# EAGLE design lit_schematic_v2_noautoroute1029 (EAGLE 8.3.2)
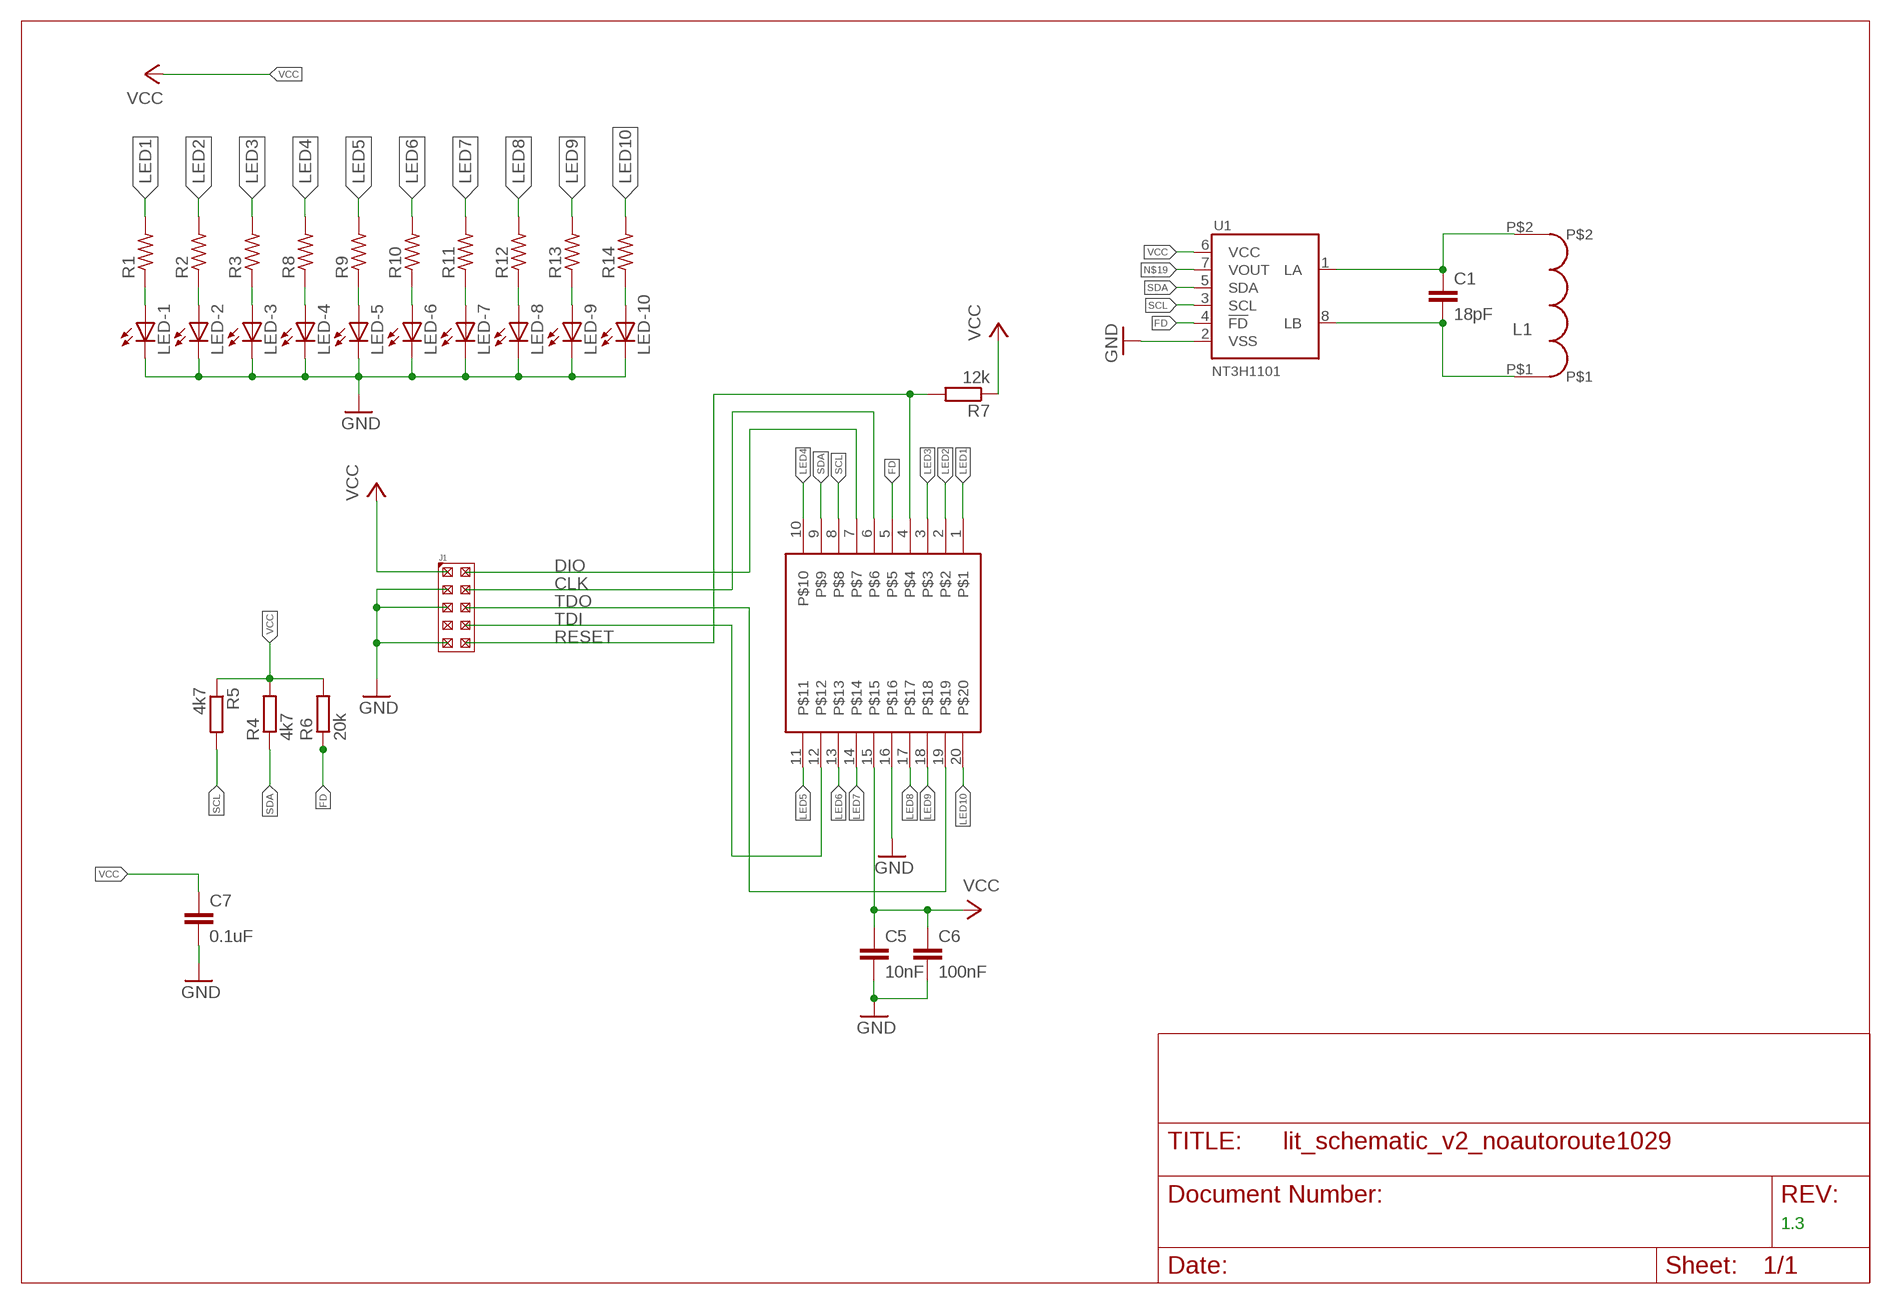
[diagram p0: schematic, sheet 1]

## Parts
C1  18pF  C-EUC0402K  [C0402K]
C5  10nF  C-EUC0402K  [C0402K]
C6  100nF  C-EUC0402K  [C0402K]
C7  0.1uF  C-EUC0402K  [C0402K]
J1  J-10-2X5_B0D95-10  [BD095-10]
L1  NXP_PICC_ANTENNAS_TEST_CLASS_05_50PF_01  [NXP_PICC_ANTENNAS_TEST_L_PICC_CLASS5_50PF_01]
LED-1  LEDCHIPLED_1206  [CHIPLED_1206]
LED-2  LEDCHIPLED_1206  [CHIPLED_1206]
LED-3  LEDCHIPLED_1206  [CHIPLED_1206]
LED-4  LEDCHIPLED_1206  [CHIPLED_1206]
LED-5  LEDCHIPLED_1206  [CHIPLED_1206]
LED-6  LEDCHIPLED_1206  [CHIPLED_1206]
LED-7  LEDCHIPLED_1206  [CHIPLED_1206]
LED-8  LEDCHIPLED_1206  [CHIPLED_1206]
LED-9  LEDCHIPLED_1206  [CHIPLED_1206]
LED-10  LEDCHIPLED_1206  [CHIPLED_1206]
R1  R-US_R0402  [R0402]
R2  R-US_R0402  [R0402]
R3  R-US_R0402  [R0402]
R4  4k7  R-EU_R0402  [R0402]
R5  4k7  R-EU_R0402  [R0402]
R6  20k  R-EU_R0402  [R0402]
R7  12k  R-EU_R0402  [R0402]
R8  R-US_R0402  [R0402]
R9  R-US_R0402  [R0402]
R10  R-US_R0402  [R0402]
R11  R-US_R0402  [R0402]
R12  R-US_R0402  [R0402]
R13  R-US_R0402  [R0402]
R14  R-US_R0402  [R0402]
U1  NT3H1101  [TSSOP8]
U$1  LPC812  NXP_LPC80012_TSSOP20  [TSSOP20]

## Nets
CLK: J1.P$4 U$1.6
DIO: J1.P$2 U$1.7
FD: R6.1 U1.4(!FD) U$1.5
GND: C5.2 C6.2 C7.2 J1.P$3 J1.P$5 J1.P$9 LED-1.C LED-2.C LED-3.C LED-4.C LED-5.C LED-6.C LED-7.C LED-8.C LED-9.C LED-10.C U1.2(VSS) U$1.16
LED1: R1.2 U$1.1
LED2: R2.2 U$1.2
LED3: R3.2 U$1.3
LED4: R8.2 U$1.10
LED5: R9.2 U$1.11
LED6: R10.2 U$1.13
LED7: R11.2 U$1.14
LED8: R12.2 U$1.17
LED9: R13.2 U$1.18
LED10: R14.2 U$1.20
N$1: C1.2 L1.P$1 U1.8(LB)
N$2: LED-1.A R1.1
N$3: LED-2.A R2.1
N$4: LED-3.A R3.1
N$5: LED-4.A R8.1
N$6: LED-5.A R9.1
N$7: LED-6.A R10.1
N$8: LED-7.A R11.1
N$9: LED-8.A R12.1
N$10: LED-9.A R13.1
N$13: C1.1 L1.P$2 U1.1(LA)
N$15: LED-10.A R14.1
N$19: U1.7(VOUT)
RESET: J1.P$10 R7.2 U$1.4
SCL: R5.2 U1.3(SCL) U$1.8
SDA: R4.1 U1.5(SDA) U$1.9
TDI: J1.P$8 U$1.12
TDO: J1.P$6 U$1.19
VCC: C5.1 C6.1 C7.1 J1.P$1 R4.2 R5.1 R6.2 R7.1 U1.6(VCC) U$1.15
Unconnected: J1.P$7

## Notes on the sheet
- 1.3

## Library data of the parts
C1 C5-C7 = rcl:C-EU: CAPACITOR, European symbol
J1 = STL50S-10:J-10-2X5
L1 = NTag_I2C_Class5_V5:NXP_PICC_ANTENNAS_TEST_CLASS_05_50PF_01: Class 5 Antenna - 50 pF #01
LED-1-LED-10 = led:LED: LED
R1-R3 R8-R14 = resistor:R-US_: RESISTOR, American symbol
R4-R7 = rcl:R-EU_: RESISTOR, European symbol
U1 = NXP_60_26022015:NT3H1101: NTAG I²C, NFC Forum type 2 Tag compliant IC with I²C interface The NTAG I2C is the first product of NXP’s NTAG family offering both contactless and contact interfaces (see Figure 1). In addition to the passive NFC Forum compliant contactless interface, the IC features an I²C contact interface,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
U$1 = stefan_ref-packages-longpad:NXP_LPC80012_TSSOP20

## Module TEST
Ports: PORT(io)

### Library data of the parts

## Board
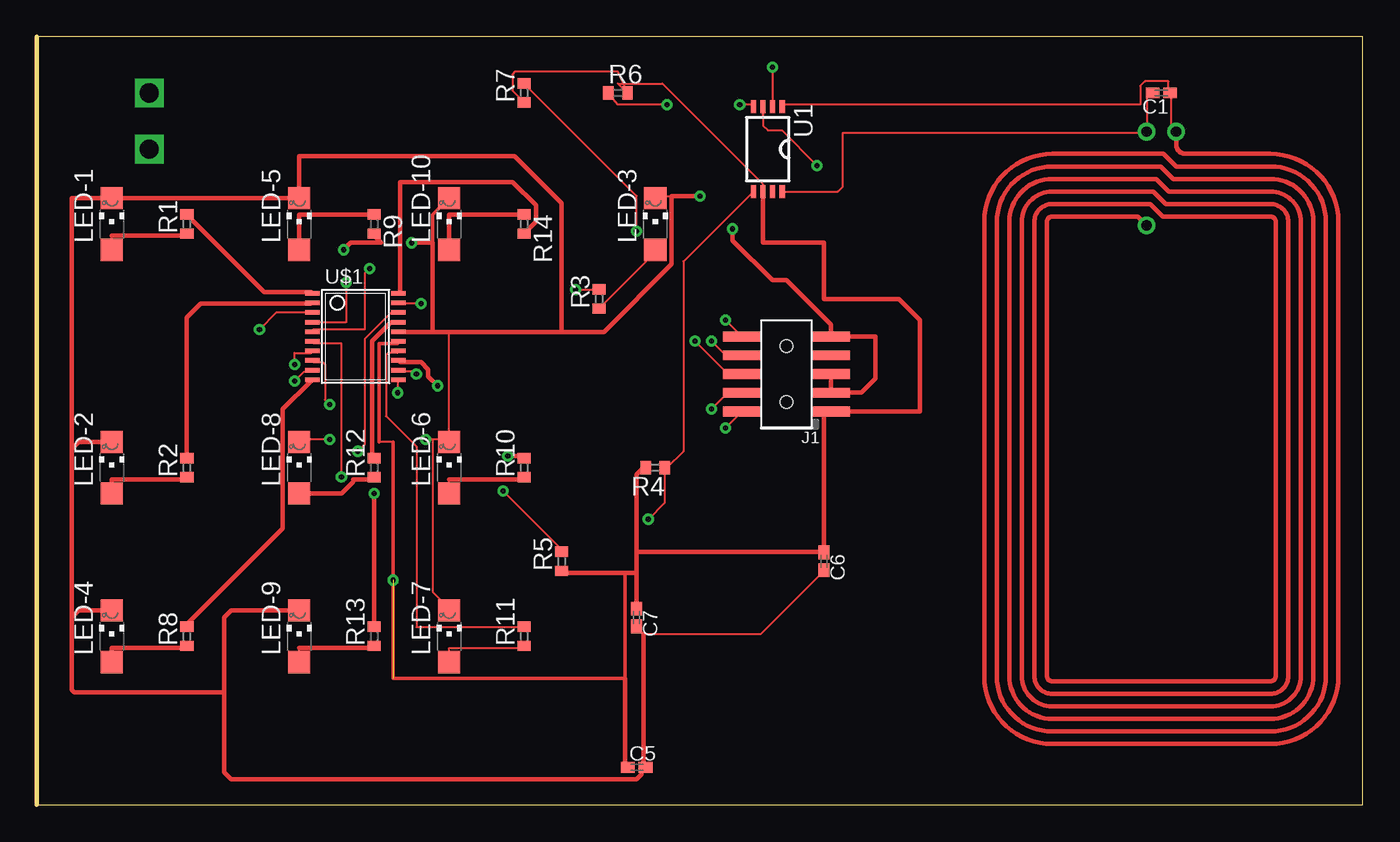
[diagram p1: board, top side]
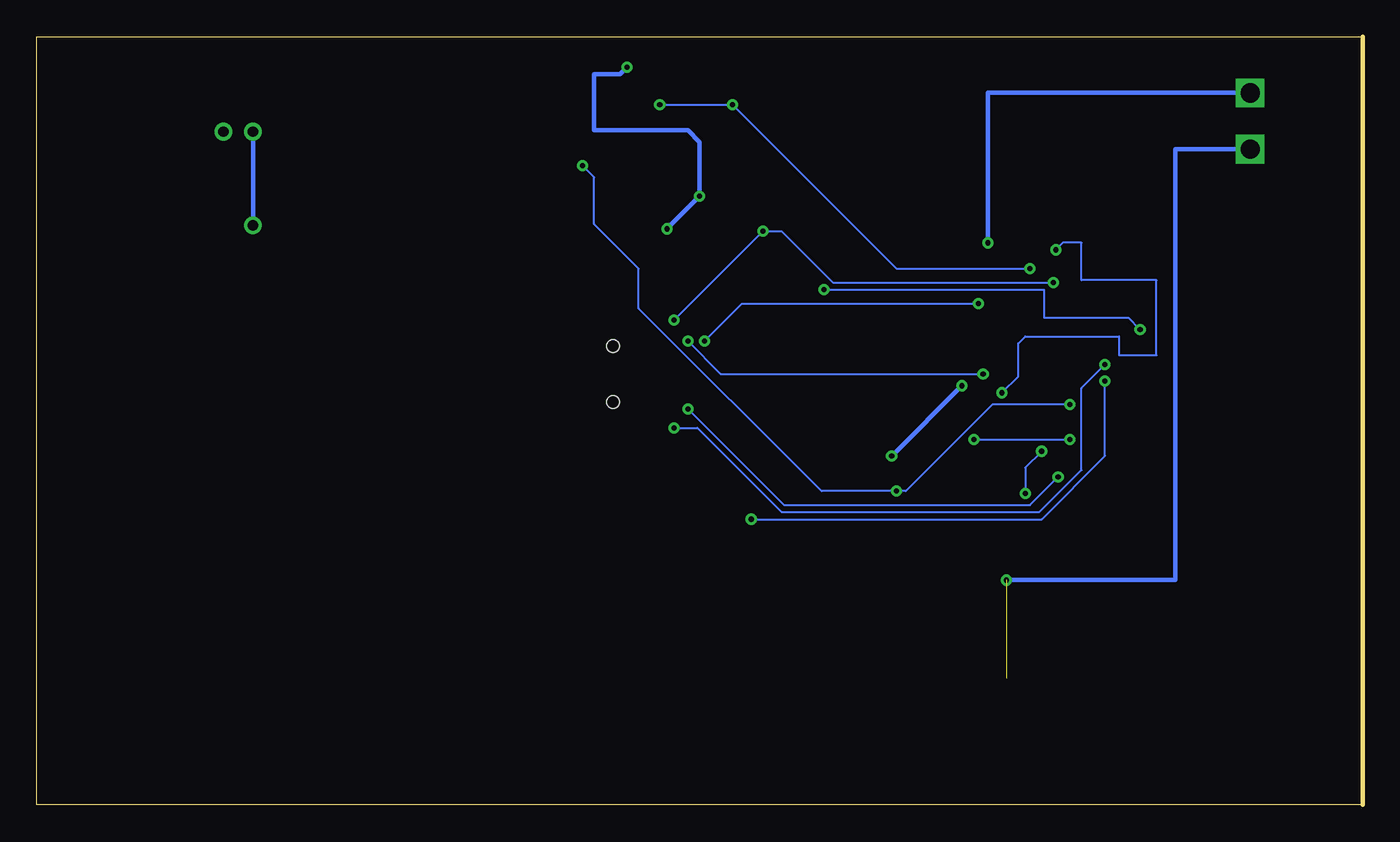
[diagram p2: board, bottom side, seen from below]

Size 89.84 x 52.06 mm. Coordinates in mm from the lower left corner, seen from the top.
Outline: 0,0 89.84,0 89.84,52.06 0,52.06 0,0
Copper layers (1*16): Top 0.035mm / dielectric 1.5mm / Bottom 0.035mm
Design rules "default *": minimum track width 6mil, minimum drill 0.35mm, track to track 6mil, track to pad 6mil, pad to pad 6mil, via to via 6mil, smd to smd 10mil, copper to edge 40mil, drill to drill 6mil, minimum pad ring 10mil, minimum via ring 8mil, stop-mask expansion 4mil, vias tented up to drill 0mil, thermal gap 10mil

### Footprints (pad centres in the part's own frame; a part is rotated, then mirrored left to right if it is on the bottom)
C0402K = smd 0.925 x 0.74: 1 -0.6,0; 2 0.6,0
BD095-10 = smd 0.65 x 2.6: P$1 -2.54,-3; P$2 -2.54,3; P$3 -1.27,-3; P$4 -1.27,3; P$5 0,-3; P$6 0,3; P$7 1.27,-3; P$8 1.27,3; P$9 2.54,-3; P$10 2.54,3 | hole 0.85: 1.905,0; -1.905,0
NXP_PICC_ANTENNAS_TEST_L_PICC_CLASS5_50PF_01 = drill 0.7: P$1 21.5,1; P$2 21.5,-1; P$3 15.15,1
CHIPLED_1206 = smd 1.5 x 1.5: A 0,-1.75; C 0,1.75
R0402 = smd 0.7 x 0.9: 1 -0.65,0; 2 0.65,0
TSSOP8 = smd 0.9 x 0.35: 1 -2.875,0.975; 2 -2.875,0.325; 3 -2.875,-0.325; 4 -2.875,-0.975; 5 2.875,-0.975; 6 2.875,-0.325; 7 2.875,0.325; 8 2.875,0.975
TSSOP20 = smd 0.305 x 0.991: 1 -2.925,-2.918; 2 -2.275,-2.918; 3 -1.625,-2.918; 4 -0.975,-2.918; 5 -0.325,-2.918; 6 0.325,-2.918; 7 0.975,-2.918; 8 1.625,-2.918; 9 2.275,-2.918; 10 2.925,-2.918; 11 2.925,2.918; 12 2.275,2.918; 13 1.625,2.918; 14 0.975,2.918; 15 0.325,2.918; 16 -0.325,2.918; 17 -0.975,2.918; 18 -1.625,2.918; 19 -2.275,2.918; 20 -2.925,2.918

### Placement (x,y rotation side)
C1  76.2,48.26 180 top
C5  40.64,2.54 0 top
C6  53.34,16.51 270 top
C7  40.64,12.7 270 top
J1  50.8,29.21 90 top
L1  76.2,24.13 90 top
LED-1  5.08,39.37 0 top
LED-2  5.08,22.86 0 top
LED-3  41.91,39.37 0 top
LED-4  5.08,11.43 0 top
LED-5  17.78,39.37 0 top
LED-6  27.94,22.86 0 top
LED-7  27.94,11.43 0 top
LED-8  17.78,22.86 0 top
LED-9  17.78,11.43 0 top
LED-10  27.94,39.37 0 top
R1  10.16,39.37 90 top
R2  10.16,22.86 90 top
R3  38.1,34.29 90 top
R4  41.91,22.86 180 top
R5  35.56,16.51 90 top
R6  39.37,48.26 0 top
R7  33.02,48.26 90 top
R8  10.16,11.43 90 top
R9  22.86,39.37 270 top
R10  33.02,22.86 90 top
R11  33.02,11.43 90 top
R12  22.86,22.86 90 top
R13  22.86,11.43 90 top
R14  33.02,39.37 270 top
U1  49.53,44.45 270 top
U$1  21.59,31.75 270 top

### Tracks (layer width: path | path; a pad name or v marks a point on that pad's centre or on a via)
CLK  (via drill 0.35)
  Top 0.152: v20.64,22.23 20.64,31.27 18.73,31.27 U$1.6 | v45.72,26.83 46.83,27.94 J1.P$4
  Bottom 0.152: v20.64,22.23 22.54,20.32 39.21,20.32 v45.72,26.83
DIO  (via drill 0.35)
  Top 0.152: v17.46,29.84 17.46,30.64 18.57,30.64 U$1.7 | v46.67,25.56 47.78,26.67 J1.P$2
  Bottom 0.152: v17.46,29.84 19.05,28.26 19.05,22.7 21.91,19.84 39.37,19.84 45.09,25.56 v46.67,25.56
FD  (via drill 0.35)
  Top 0.152: v42.7,47.47 39.37,47.47 R6.1 | v47.62,47.47 48.42,47.47 U1.4 | v22.54,36.35 22.22,36.04 22.22,32.23 18.73,32.23 U$1.5
  Bottom 0.152: v47.62,47.47 v42.7,47.47 31.59,36.35 v22.54,36.35
GND  (via drill 0.35, 1.3)
  Top 0.152: 53.82,29.21 J1.P$5 | v49.85,50.01 49.85,47.31 U1.2 | 43.02,41.27 41.91,41.27 LED-3.C | 53.66,31.75 J1.P$9 | 27.94,24.77 27.94,32.07 | 24.61,32.07 U$1.16 | v19.84,24.77 17.78,24.77 LED-8.C | 27.94,24.77 26.83,24.77 | 26.83,24.77 v26.35,24.77 | 27.94,24.77 LED-6.C | 26.83,24.77 26.83,14.45 27.94,13.34 LED-7.C | LED-10.C | C7.2 40.64,12.06 41.12,11.59 49.05,11.59 53.34,15.88 C6.2 | LED-5.C | 5.08,13.34 LED-4.C | LED-2.C | LED-9.C | LED-1.C | 40.96,2.38 41.12,2.54 C5.2 | 53.82,28.26 53.82,27.94 J1.P$3 53.82,28.26
  Top 0.254: LED-10.C 26.83,40.01 26.83,38.1
  Top 0.305: 53.82,29.21 53.82,28.26 | v44.93,41.27 43.02,41.27 43.02,36.67 38.42,32.07 35.56,32.07 | v47.15,39.05 47.15,38.26 49.85,35.56 50.8,35.56 53.8,32.56 J1.P$9 56.83,31.75 56.83,28.89 55.88,27.94 J1.P$3 | 26.83,32.07 27.94,32.07 35.56,32.07 | 26.83,32.07 24.61,32.07 | 26.83,32.07 26.83,38.1 v25.4,38.1 | 41.12,2.54 41.12,11.59 | LED-5.C LED-1.C | 40.96,2.38 40.96,2.06 40.64,1.75 13.18,1.75 12.7,2.22 12.7,7.62 | 35.56,32.07 35.56,40.8 32.38,43.97 17.78,43.97 LED-5.C | LED-1.C 2.36,41.12 2.36,24.13 | 2.36,24.13 2.36,12.7 | 2.36,12.7 2.36,7.8 2.54,7.62 12.7,7.62 | LED-4.C 2.84,13.18 2.36,12.7 | LED-2.C 2.84,24.61 2.36,24.13 | LED-9.C 13.18,13.18 12.7,12.7 12.7,7.62
  Bottom 0.152: v26.35,24.77 v19.84,24.77
  Bottom 0.305: v47.15,39.05 v44.93,41.27 44.93,44.93 45.72,45.72 52.07,45.72 52.07,49.53 50.32,49.53 v49.85,50.01 | v25.4,38.1 25.4,48.26 v7.62,48.26
LED1
  Top 0.152: 10.16,40.01 R1.2 | 18.57,34.77 U$1.1
  Top 0.305: 10.16,40.01 15.4,34.77 18.57,34.77
LED2
  Top 0.152: U$1.2 18.57,33.97
  Top 0.305: 18.57,33.97 11.11,33.97 10.16,33.02 R2.2
LED3  (via drill 0.35)
  Top 0.152: v36.51,34.92 38.1,34.92 R3.2 | 18.73,33.5 U$1.3 16.23,33.38 v15.08,32.23
  Bottom 0.152: v36.51,34.92 21.59,34.92 21.59,33.02 15.88,33.02 v15.08,32.23
LED4
  Top 0.152: 10.16,12.22 R8.2 | 18.57,28.73 U$1.10
  Top 0.305: 10.16,12.22 16.67,18.73 16.67,26.83 18.57,28.73
LED5  (via drill 0.35)
  Top 0.152: v24.45,27.94 24.45,28.73 U$1.11 | 22.86,38.58 R9.2
  Top 0.305: 22.86,38.58 23.34,38.1 21.27,38.1 v20.8,37.62
  Bottom 0.152: v24.45,27.94 23.34,29.05 23.34,31.27 22.86,31.75 16.51,31.75 16.51,30.48 13.97,30.48 13.97,35.56 19.05,35.56 19.05,38.1 20.32,38.1 v20.8,37.62
LED6  (via drill 0.35)
  Top 0.152: 33.02,23.65 R10.2 | 24.61,30 U$1.13
  Top 0.305: v31.91,23.65 33.02,23.65 | v27.15,28.42 26.51,29.05 26.51,29.53 26.04,30 24.61,30
  Bottom 0.305: v27.15,28.42 v31.91,23.65
LED7
  Top 0.152: R11.2 33.02,12.06 25.72,12.06 25.72,24.29 23.65,26.35 23.65,30.48 23.81,30.64 24.45,30.64 U$1.14
LED8
  Top 0.152: 22.7,23.81 22.86,23.65 R12.2 | 23.97,32.7 24.45,32.7 U$1.17
  Top 0.305: 22.7,23.81 22.7,31.43 23.97,32.7
LED9  (via drill 0.35)
  Top 0.152: v21.75,23.97 22.22,24.45 22.22,31.59 23.97,33.34 24.45,33.34 U$1.18
  Top 0.305: v22.86,21.11 R13.2
  Bottom 0.152: v22.86,21.11 22.86,22.86 v21.75,23.97
LED10
  Top 0.152: 33.02,38.73 R14.2 | 24.61,34.77 U$1.20
  Top 0.305: 33.02,38.73 33.81,39.53 33.81,40.64 32.23,42.23 24.61,42.23 24.61,34.77
N$1
  Top 0.152: 50.64,41.59 U1.8 54.28,41.58 54.61,41.91 54.61,45.56 75.09,45.56 L1.P$1 75.25,45.72 75.25,47.94 75.56,48.26 C1.2
N$2
  Top 0.152: LED-1.A 5.08,38.58 | 10.16,38.58 R1.1
  Top 0.305: 5.08,38.58 10.16,38.58
N$3
  Top 0.152: 10.16,22.07 R2.1
  Top 0.305: 10.16,22.07 5.08,22.07 LED-2.A
N$4
  Top 0.152: R3.1 38.1,33.66 41.91,37.47 LED-3.A
N$5
  Top 0.152: 10.16,10.64 R8.1
  Top 0.305: 10.16,10.64 5.08,10.64 LED-4.A
N$6
  Top 0.152: 22.86,40.01 R9.1
  Top 0.305: 22.86,40.01 17.78,40.01 LED-5.A
N$7
  Top 0.152: LED-6.A 27.94,22.07 | 33.02,22.07 R10.1
  Top 0.305: 27.94,22.07 33.02,22.07
N$8
  Top 0.152: LED-7.A 27.94,10.64 33.02,10.64 R11.1
N$9
  Top 0.152: 21.43,21.91 21.43,22.07 | 22.86,22.07 R12.1 | LED-8.A
  Top 0.305: 21.43,22.07 22.86,22.07 | 21.43,21.91 20.64,21.11 LED-8.A
N$10
  Top 0.152: LED-9.A 17.78,10.64 | 22.86,10.64 R13.1
  Top 0.305: 17.78,10.64 22.86,10.64
N$13
  Top 0.152: U1.1 50.64,47.47 74.77,47.47 74.77,48.74 75.09,49.05 76.68,49.05 76.68,48.26 C1.1 76.83,48.26 76.83,46.04 77.15,45.72 L1.P$2
N$15
  Top 0.152: 33.02,40.01 R14.1
  Top 0.305: 33.02,40.01 27.94,40.01 LED-10.A
RESET  (via drill 0.35)
  Top 0.152: v40.64,38.89 40.64,41.27 33.02,48.9 R7.2 | v46.67,32.86 47.78,31.75 J1.P$10 | v20.95,35.4 20.95,32.7 18.73,32.7 U$1.4
  Bottom 0.152: v46.67,32.86 v40.64,38.89 39.37,38.89 35.88,35.4 v20.95,35.4
SCL  (via drill 0.35)
  Top 0.152: v31.59,21.27 35.56,17.3 R5.2 | v19.84,27.15 19.53,27.46 19.53,29.84 19.37,30 18.73,30 U$1.8 | 49.21,46.67 49.21,46.99 | 49.21,46.99 49.21,47.31 U1.3 | 49.21,46.99 49.21,46.04 49.53,45.72 50.48,45.72 v52.86,43.34
  Bottom 0.152: v19.84,27.15 25.08,27.15 30.96,21.27 v31.59,21.27 36.67,21.27 49.05,33.66 49.05,36.35 52.07,39.37 52.07,42.55 v52.86,43.34
SDA  (via drill 0.35)
  Top 0.152: U1.5 48.42,41.43 43.82,36.83 43.82,23.97 42.7,22.86 R4.1 42.55,22.86 42.55,20.48 v41.43,19.37 | v17.46,28.73 18.1,29.37 18.57,29.37 U$1.9
  Bottom 0.152: v17.46,28.73 17.46,23.65 21.75,19.37 v41.43,19.37
TDI  (via drill 0.35)
  Top 0.152: v25.72,29.21 25.72,29.37 24.61,29.37 U$1.12 | v45.72,31.43 46.67,30.48 J1.P$8
  Bottom 0.152: v25.72,29.21 43.5,29.21 v45.72,31.43
TDO  (via drill 0.35)
  Top 0.152: v26.04,33.97 24.61,33.97 U$1.19 | v44.61,31.43 46.83,29.21 J1.P$6
  Bottom 0.152: v26.04,33.97 42.07,33.97 v44.61,31.43
VCC  (via drill 0.35, 1.3)  (1 unrouted)
  Top 0.152: R7.1 33.02,47.62 32.23,48.42 32.23,49.53 32.38,49.69 39.37,49.69 R6.2 39.37,48.9 42.39,48.9 49.21,42.07 49.21,41.59 U1.6 49.21,41.43 | J1.P$1 53.66,26.67 53.34,26.35 | 35.56,15.72 R5.1 | 41.12,22.86 R4.2 | 39.85,2.7 40.01,2.54 C5.1 | 24.45,31.27 U$1.15 | 53.34,17.14 C6.1 | 24.13,24.61 23.18,24.61
  Top 0.254: 39.85,15.72 39.85,8.57 24.13,8.57 24.13,24.61 | 24.45,31.27 23.18,31.27 23.18,24.61
  Top 0.305: 40.64,15.72 39.85,15.72 35.56,15.72 | C7.1 40.64,15.72 | 41.12,22.86 40.64,22.38 40.64,17.14 | 40.64,15.72 40.64,17.14 | 39.85,8.57 39.85,2.7 | 40.64,17.14 53.34,17.14 | C6.1 53.34,26.35 | J1.P$1 59.85,26.67 59.85,32.86 58.42,34.29 53.34,34.29 53.34,38.1 49.21,38.1 U1.6
  Bottom 0.305: v24.13,15.24 12.7,15.24 12.7,44.45 v7.62,44.45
